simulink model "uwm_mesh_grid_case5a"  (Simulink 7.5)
settings: Solver=ode45  StartTime=0.0  StopTime=3.0  RelTol=1e-4
undefined symbols (not defined in the file or in its folder): D1, Delta, dfilt, DiscIntNeverNeededParam, Discrete, no, powergui, steady, ZData
libraries: powerlib x259, powerlib_extras x68, dsparch4 x11
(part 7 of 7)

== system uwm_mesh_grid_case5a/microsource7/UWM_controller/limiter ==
  In1 : Inport
  Integrator1 : Integrator  LimitOutput=on  UpperSaturationLimit=0  LowerSaturationLimit=-pi  ZeroCross=off
  Integrator2 : Integrator  LimitOutput=on  UpperSaturationLimit=pi  LowerSaturationLimit=0  ZeroCross=off
  Kilim : Gain  Gain=30  ParameterDataType=sfix(16)  ParameterScaling=2^0  OutDataType=sfix(16)  OutScaling=2^0
  Kilim1 : Gain  Gain=30  ParameterDataType=sfix(16)  ParameterScaling=2^0  OutDataType=sfix(16)  OutScaling=2^0
  Kplim : Gain  Gain=3  ParameterDataType=sfix(16)  ParameterScaling=2^0  OutDataType=sfix(16)  OutScaling=2^0
  Kplim1 : Gain  Gain=3  ParameterDataType=sfix(16)  ParameterScaling=2^0  OutDataType=sfix(16)  OutScaling=2^0
  Plimit : Constant  Value=1.0  OutDataType=sfix(16)  OutScaling=2^0
  Plimit1 : Constant  Value=0.0  OutDataType=sfix(16)  OutScaling=2^0
  Saturation1 : Saturate  UpperLimit=pi  LowerLimit=0  OutDataType=fixdt(1, 16)  OutScaling=2^0
  Saturation2 : Saturate  UpperLimit=0  LowerLimit=-pi  OutDataType=fixdt(1, 16)  OutScaling=2^0
  Sum1 : Sum  Inputs=-+|  OutDataType=sfix(16)  OutScaling=2^0
  Sum2 : Sum  Inputs=|++  OutDataType=sfix(16)  OutScaling=2^0
  Sum3 : Sum  OutDataType=sfix(16)  OutScaling=2^0
  Sum4 : Sum  Inputs=|+-  OutDataType=sfix(16)  OutScaling=2^0
  Sum9 : Sum  Inputs=|++  OutDataType=sfix(16)  OutScaling=2^0
  Out1 : Outport
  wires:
  Sum3/1 -> Out1/1
  Plimit1/1 -> Sum1/2
  Integrator2/1 -> Sum2/2
  Kilim1/1 -> Integrator2/1
  Sum1/1 -> Kilim1/1, Kplim1/1
  In1/1 -> Sum1/1, Sum4/2
  Integrator1/1 -> Sum9/2
  Kilim/1 -> Integrator1/1
  Sum4/1 -> Kilim/1, Kplim/1
  Plimit/1 -> Sum4/1
  Kplim1/1 -> Saturation1/1
  Saturation1/1 -> Sum2/1
  Kplim/1 -> Saturation2/1
  Saturation2/1 -> Sum9/1
  Sum9/1 -> Sum3/1
  Sum2/1 -> Sum3/2

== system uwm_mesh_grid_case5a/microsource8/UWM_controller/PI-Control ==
  In1 : Inport
  Gain : Gain  Gain=.01  ParameterDataType=sfix(16)  ParameterScaling=2^0  OutDataType=sfix(16)  OutScaling=2^0
  Gain1 : Gain  Gain=5  ParameterDataType=sfix(16)  ParameterScaling=2^0  OutDataType=sfix(16)  OutScaling=2^0
  Gain2 : Gain  Gain=750  ParameterDataType=sfix(16)  ParameterScaling=2^0  OutDataType=sfix(16)  OutScaling=2^0
  Integrator1 : Integrator  LimitOutput=on  UpperSaturationLimit=100  LowerSaturationLimit=-100  ZeroCross=off
  Sum4 : Sum  Inputs=|++  OutDataType=sfix(16)  OutScaling=2^0
  Out1 : Outport
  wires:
  Gain/1 -> Sum4/1
  Integrator1/1 -> Sum4/2
  In1/1 -> Gain1/1, Gain/1
  Gain1/1 -> Integrator1/1
  Sum4/1 -> Gain2/1
  Gain2/1 -> Out1/1

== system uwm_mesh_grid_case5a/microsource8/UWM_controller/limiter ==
  In1 : Inport
  Integrator1 : Integrator  LimitOutput=on  UpperSaturationLimit=0  LowerSaturationLimit=-pi  ZeroCross=off
  Integrator2 : Integrator  LimitOutput=on  UpperSaturationLimit=pi  LowerSaturationLimit=0  ZeroCross=off
  Kilim : Gain  Gain=30  ParameterDataType=sfix(16)  ParameterScaling=2^0  OutDataType=sfix(16)  OutScaling=2^0
  Kilim1 : Gain  Gain=30  ParameterDataType=sfix(16)  ParameterScaling=2^0  OutDataType=sfix(16)  OutScaling=2^0
  Kplim : Gain  Gain=3  ParameterDataType=sfix(16)  ParameterScaling=2^0  OutDataType=sfix(16)  OutScaling=2^0
  Kplim1 : Gain  Gain=3  ParameterDataType=sfix(16)  ParameterScaling=2^0  OutDataType=sfix(16)  OutScaling=2^0
  Plimit : Constant  Value=1.0  OutDataType=sfix(16)  OutScaling=2^0
  Plimit1 : Constant  Value=0.0  OutDataType=sfix(16)  OutScaling=2^0
  Saturation1 : Saturate  UpperLimit=pi  LowerLimit=0  OutDataType=fixdt(1, 16)  OutScaling=2^0
  Saturation2 : Saturate  UpperLimit=0  LowerLimit=-pi  OutDataType=fixdt(1, 16)  OutScaling=2^0
  Sum1 : Sum  Inputs=-+|  OutDataType=sfix(16)  OutScaling=2^0
  Sum2 : Sum  Inputs=|++  OutDataType=sfix(16)  OutScaling=2^0
  Sum3 : Sum  OutDataType=sfix(16)  OutScaling=2^0
  Sum4 : Sum  Inputs=|+-  OutDataType=sfix(16)  OutScaling=2^0
  Sum9 : Sum  Inputs=|++  OutDataType=sfix(16)  OutScaling=2^0
  Out1 : Outport
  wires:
  Sum3/1 -> Out1/1
  Plimit1/1 -> Sum1/2
  Integrator2/1 -> Sum2/2
  Kilim1/1 -> Integrator2/1
  Sum1/1 -> Kilim1/1, Kplim1/1
  In1/1 -> Sum1/1, Sum4/2
  Integrator1/1 -> Sum9/2
  Kilim/1 -> Integrator1/1
  Sum4/1 -> Kilim/1, Kplim/1
  Plimit/1 -> Sum4/1
  Kplim1/1 -> Saturation1/1
  Saturation1/1 -> Sum2/1
  Kplim/1 -> Saturation2/1
  Saturation2/1 -> Sum9/1
  Sum9/1 -> Sum3/1
  Sum2/1 -> Sum3/2

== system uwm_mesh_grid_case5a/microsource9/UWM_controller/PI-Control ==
  In1 : Inport
  Gain : Gain  Gain=.01  ParameterDataType=sfix(16)  ParameterScaling=2^0  OutDataType=sfix(16)  OutScaling=2^0
  Gain1 : Gain  Gain=5  ParameterDataType=sfix(16)  ParameterScaling=2^0  OutDataType=sfix(16)  OutScaling=2^0
  Gain2 : Gain  Gain=750  ParameterDataType=sfix(16)  ParameterScaling=2^0  OutDataType=sfix(16)  OutScaling=2^0
  Integrator1 : Integrator  LimitOutput=on  UpperSaturationLimit=100  LowerSaturationLimit=-100  ZeroCross=off
  Sum4 : Sum  Inputs=|++  OutDataType=sfix(16)  OutScaling=2^0
  Out1 : Outport
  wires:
  Gain/1 -> Sum4/1
  Integrator1/1 -> Sum4/2
  In1/1 -> Gain1/1, Gain/1
  Gain1/1 -> Integrator1/1
  Sum4/1 -> Gain2/1
  Gain2/1 -> Out1/1

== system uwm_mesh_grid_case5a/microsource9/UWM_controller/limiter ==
  In1 : Inport
  Integrator1 : Integrator  LimitOutput=on  UpperSaturationLimit=0  LowerSaturationLimit=-pi  ZeroCross=off
  Integrator2 : Integrator  LimitOutput=on  UpperSaturationLimit=pi  LowerSaturationLimit=0  ZeroCross=off
  Kilim : Gain  Gain=30  ParameterDataType=sfix(16)  ParameterScaling=2^0  OutDataType=sfix(16)  OutScaling=2^0
  Kilim1 : Gain  Gain=30  ParameterDataType=sfix(16)  ParameterScaling=2^0  OutDataType=sfix(16)  OutScaling=2^0
  Kplim : Gain  Gain=3  ParameterDataType=sfix(16)  ParameterScaling=2^0  OutDataType=sfix(16)  OutScaling=2^0
  Kplim1 : Gain  Gain=3  ParameterDataType=sfix(16)  ParameterScaling=2^0  OutDataType=sfix(16)  OutScaling=2^0
  Plimit : Constant  Value=1.0  OutDataType=sfix(16)  OutScaling=2^0
  Plimit1 : Constant  Value=0.0  OutDataType=sfix(16)  OutScaling=2^0
  Saturation1 : Saturate  UpperLimit=pi  LowerLimit=0  OutDataType=fixdt(1, 16)  OutScaling=2^0
  Saturation2 : Saturate  UpperLimit=0  LowerLimit=-pi  OutDataType=fixdt(1, 16)  OutScaling=2^0
  Sum1 : Sum  Inputs=-+|  OutDataType=sfix(16)  OutScaling=2^0
  Sum2 : Sum  Inputs=|++  OutDataType=sfix(16)  OutScaling=2^0
  Sum3 : Sum  OutDataType=sfix(16)  OutScaling=2^0
  Sum4 : Sum  Inputs=|+-  OutDataType=sfix(16)  OutScaling=2^0
  Sum9 : Sum  Inputs=|++  OutDataType=sfix(16)  OutScaling=2^0
  Out1 : Outport
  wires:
  Sum3/1 -> Out1/1
  Plimit1/1 -> Sum1/2
  Integrator2/1 -> Sum2/2
  Kilim1/1 -> Integrator2/1
  Sum1/1 -> Kilim1/1, Kplim1/1
  In1/1 -> Sum1/1, Sum4/2
  Integrator1/1 -> Sum9/2
  Kilim/1 -> Integrator1/1
  Sum4/1 -> Kilim/1, Kplim/1
  Plimit/1 -> Sum4/1
  Kplim1/1 -> Saturation1/1
  Saturation1/1 -> Sum2/1
  Kplim/1 -> Saturation2/1
  Saturation2/1 -> Sum9/1
  Sum9/1 -> Sum3/1
  Sum2/1 -> Sum3/2

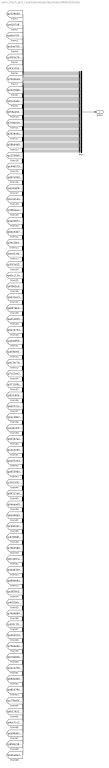
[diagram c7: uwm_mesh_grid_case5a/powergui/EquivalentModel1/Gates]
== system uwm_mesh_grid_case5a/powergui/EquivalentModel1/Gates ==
  Mux : Mux  Inputs=[1 1 1 1 1 1 1 1 1 1 1 1 1 1 1 1 1 1 1 1 1 1 1 1 1 1 1 1 1 1 1 1 1 1 1 1 1 1 1 1 1 1 1 1 1 1 1 1 1 1 1 1 1 1 1 1 1 1 1 1 1 1 1 1 1 1 1 1 1]
  gates : Outport  OutDataType=sfix(16)  OutScaling=2^0
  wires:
  Mux/1 -> gates/1
  [tpe228b584_b106_4beb_8c86_c7c8c8351509] -> Mux/1
  [tpef207a81_30da_459f_9f29_48d5e080c51c] -> Mux/2
  [tpa6e07f33_604f_4639_95d3_65b3053db820] -> Mux/3
  [tpe3ee7652_0b4f_4b52_a6a2_6f5b020b198a] -> Mux/4
  [tp3f93a760_c478_4b19_8b9a_602eaec045ba] -> Mux/5
  [tpfce110a4_06b3_4449_bb13_54bd1c524869] -> Mux/6
  [tp7024ba96_b1e0_402b_98ae_915e2eb8f599] -> Mux/7
  [tp20376989_e36f_4dba_9928_f99e877ec3f8] -> Mux/8
  [tp0ce2ade4_fe95_468c_8653_25d67a2f6720] -> Mux/9
  [tpf56e2625_fa7f_43eb_b96b_8aa41f0e0eb0] -> Mux/10
  [tp7c8d1b9a_a0ac_4205_9121_39a3ef8997d4] -> Mux/11
  [tp2628d4ad_802e_4e1e_86c6_7d3f78e79741] -> Mux/12
  [tp58b64b92_acf2_4221_8757_7d28af085dd6] -> Mux/13
  [tpc5536b6e_0140_4226_96f4_1f886dbf2188] -> Mux/14
  [tpc446579b_ad45_4666_855e_414268daf5d6] -> Mux/15
  [tpd07e0087_c4a6_4b78_9156_ac2b3f1b5b6f] -> Mux/16
  [tpda5a6f64_d918_47c0_b755_b8f491cd819e] -> Mux/17
  [tp5c2e14aa_08b7_47f7_8143_25f87816b941] -> Mux/18
  [tp79bdace3_b7b0_4249_b087_69f27f13bbc9] -> Mux/19
  [tp4a02671c_43fe_4e01_980c_0eab1f5b6319] -> Mux/20
  [tp0deddd7d_a945_4a8b_8921_7258e67777da] -> Mux/21
  [tp3ec2bb15_666f_445f_a31f_f1abb802b23d] -> Mux/22
  [tpaee1afd5_2a3a_4c4e_81d1_932180aaf4cd] -> Mux/23
  [tp35f3d32d_77d0_4ec4_8380_fc1713e814fd] -> Mux/24
  [tpd5cc13b4_db93_4301_a375_bb18755ebe77] -> Mux/25
  [tpf4062e95_3443_47db_82c0_350cf0c25750] -> Mux/26
  [tp9531e23f_24be_4071_8584_f51bbd60ef4e] -> Mux/27
  [tp69f76bb8_fdbd_4204_8031_d9110d10a512] -> Mux/28
  [tpad1e850b_84d7_4b4f_84eb_080e44351dad] -> Mux/29
  [tpbb747444_63b8_44b4_b818_e0e58927764a] -> Mux/30
  [tp1b44f6bb_f2da_48c5_bb83_4960df7e179a] -> Mux/31
  [tpb5fb0f4c_cf62_4fd9_80a4_68c4b2356418] -> Mux/32
  [tpdc3ec7bb_0663_4ba0_89e4_c1c6bfdf648e] -> Mux/33
  [tp7c52ee29_3c12_4bfa_b7a2_65a1122460f4] -> Mux/34
  [tp371168cb_fc82_4ba0_b16c_c880a08d5024] -> Mux/35
  [tp62fc80bf_2011_4d5e_9be1_b2d6273b3ea2] -> Mux/36
  [tpbd0721ef_db8d_47f7_9890_7defe1fe666e] -> Mux/37
  [tp53c38974_2706_42db_94c7_ddd4e4d3b246] -> Mux/38
  [tp1a6c43fb_a676_4586_a0d1_c5ff8f0d4ae2] -> Mux/39
  [tp933b7aeb_9fdc_4218_80c6_68c9129134d2] -> Mux/40
  [tp13e31956_19c2_465e_9930_ef33d808f5d3] -> Mux/41
  [tpaa07ae4e_8a98_4286_a633_7e0dd46b920b] -> Mux/42
  [tpa65396d1_e5c2_4e4a_8dcb_8dd232d9dcff] -> Mux/43
  [tp7817f936_9030_445a_b91d_d11df62fcea4] -> Mux/44
  [tp84221b66_9ec3_426a_9c58_687200c2f280] -> Mux/45
  [tp5deead94_68b6_4323_ad82_4c4e3d7e236e] -> Mux/46
  [tp8aa98edc_83de_43f3_b92f_8a5361184f9a] -> Mux/47
  [tpc9002618_045e_4d6a_ac72_a68281a96bd7] -> Mux/48
  [tp673f69f6_82ca_4338_aa87_d59190bf68bf] -> Mux/49
  [tp7bb55887_ef87_424a_af1b_5f1901cf865a] -> Mux/50
  [tp6c446ce2_6cd8_46c3_9120_bda7217b6b5f] -> Mux/51
  [tpd4dd329b_3e2b_4ba8_9125_5a1fe0d0b51a] -> Mux/52
  [tpd69eb8ae_aeda_4526_9dd4_f402d4137f04] -> Mux/53
  [tpc605fb3f_fb8c_4d73_b613_a089dad69b67] -> Mux/54
  [tp4f07b6c9_f4fc_449c_8932_a78d658e8135] -> Mux/55
  [tp74d68840_4b65_4268_ba1a_ab971938b5e8] -> Mux/56
  [tp592c1fc9_f3c2_44fd_b305_e35d9eb2ac04] -> Mux/57
  [tpa5b5019c_88d7_4d6f_9ab7_8e2d3a81cd78] -> Mux/58
  [tp75bde6a7_ec4d_4fc1_be1b_a4b562858042] -> Mux/59
  [tp0c5bb0bd_c4ad_4771_9dea_76c1bb1f8057] -> Mux/60
  [tp2ec27d90_4684_4437_8959_f6e479ef260b] -> Mux/61
  [tpb8dbdd89_c217_41ad_bcb2_15a8ca9ae5c1] -> Mux/62
  [tpe81079eb_0f20_43dd_885d_1225b6d7928e] -> Mux/63
  [tpc79ed3fe_559f_4f8f_be41_c95cc4f1d8e1] -> Mux/64
  [tpfb178219_10dc_471f_9f4e_2f5eeda652e1] -> Mux/65
  [tp4ac7cc24_7bdd_464e_9199_ae2da14c3347] -> Mux/66
  [tpee96da57_8a75_4e0e_8896_4195514b6dd0] -> Mux/67
  [tp9f48c58f_8624_4c9f_89d7_eb94e2365c4b] -> Mux/68
  [tp52be8a3f_5ef1_470d_9c61_385db7766b04] -> Mux/69

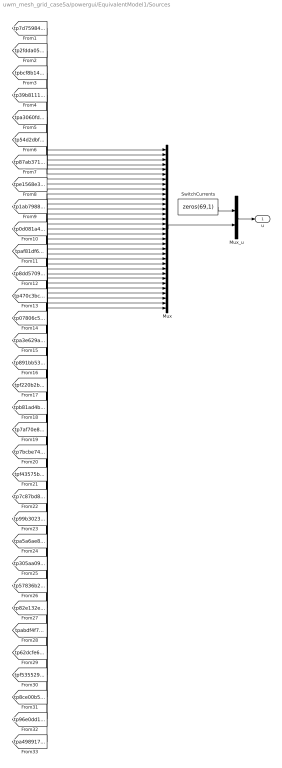
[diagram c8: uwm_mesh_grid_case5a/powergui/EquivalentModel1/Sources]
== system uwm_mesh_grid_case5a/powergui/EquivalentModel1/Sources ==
  Mux : Mux  Inputs=[2 2 1 1 1 1 1 1 1 1 1 1 1 1 1 1 1 1 1 1 1 1 1 1 1 1 1 1 1 1 1 1 3]
  Mux_u : Mux  Inputs=[69 37]
  SwitchCurrents : Constant  Value=zeros(69,1)  OutDataType=sfix(16)  OutScaling=2^0
  u : Outport  OutDataType=sfix(16)  OutScaling=2^0
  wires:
  Mux/1 -> Mux_u/2
  SwitchCurrents/1 -> Mux_u/1
  Mux_u/1 -> u/1
  [tp7d759843_31d9_4042_9dd1_9d642f5f0ff6] -> Mux/1
  [tp2fdda057_d641_4494_87e2_4c9b57d21964] -> Mux/2
  [tpbcf8b145_bdbd_45a5_8180_c3b948527696] -> Mux/3
  [tp39b81111_6fe0_4f05_ad16_780e8486a916] -> Mux/4
  [tpa3060fd9_7bb9_417d_8175_8f81b43b5773] -> Mux/5
  [tp54d2dbf4_60ce_493f_bb15_bc46fa13cfce] -> Mux/6
  [tp87ab3716_8e1d_4485_9e1a_7dc248724a34] -> Mux/7
  [tpe1568e33_bb97_4973_8708_9b1bfa17e7b5] -> Mux/8
  [tp1ab79880_228a_47d9_b201_2eba8816ee37] -> Mux/9
  [tp0d081a4d_5e9f_4b80_b4bf_20152486f853] -> Mux/10
  [tpaf81df68_c781_4da9_928a_44e197fbd618] -> Mux/11
  [tp8dd5709b_0ddf_41b6_8112_b238b0604763] -> Mux/12
  [tp470c3bc4_f7fa_46bc_9d1d_7daedd95ab4d] -> Mux/13
  [tp07806c5c_c32f_4993_b5c9_0567717f058b] -> Mux/14
  [tpa3e629a0_aa84_4358_8c69_1a4ec5cc445c] -> Mux/15
  [tp891bb538_b5bf_4ed0_b431_af5b4feecf62] -> Mux/16
  [tpf220b2bc_30ec_49dc_84aa_16925a585808] -> Mux/17
  [tpb81ad4b4_5942_43b4_8611_4a5e3db6afea] -> Mux/18
  [tp7af70e86_5434_4a0b_a65f_cb50f4951e25] -> Mux/19
  [tp7bcbe742_1608_4799_b18e_3f319801db3a] -> Mux/20
  [tpf43575be_15e6_453b_8afc_ade3ef51566d] -> Mux/21
  [tp7c87bd8b_32e3_4f6e_b2e4_4d41421fbded] -> Mux/22
  [tp99b3023c_53a1_4cb1_8eb9_8a0dd0b275b4] -> Mux/23
  [tpa5a6ae8e_c854_40e8_9ddc_396f1146314e] -> Mux/24
  [tp305aa09b_c490_428b_885a_4fbc8d6842c6] -> Mux/25
  [tp57836b25_c200_437c_8731_9b11c5d96589] -> Mux/26
  [tp82e132eb_2e2c_4493_9e5a_5b60972280db] -> Mux/27
  [tpabdf4f74_f4c9_43eb_b6bb_d288b3c0828e] -> Mux/28
  [tp62dcfe63_a088_4110_93e8_40b42f148094] -> Mux/29
  [tpf535529d_f631_44eb_ab48_591eb2ee78c0] -> Mux/30
  [tp8ce00b5d_5cb0_4337_89a4_c9ddeba94b1d] -> Mux/31
  [tp96e0dd11_cb3a_442d_8983_7206ff209956] -> Mux/32
  [tpa4989172_9284_44b3_847a_72b6f9fc12e1] -> Mux/33

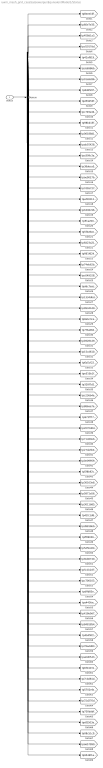
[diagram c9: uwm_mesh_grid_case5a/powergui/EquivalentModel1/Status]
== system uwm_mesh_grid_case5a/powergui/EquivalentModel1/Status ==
  status : Inport  OutDataType=sfix(16)  OutScaling=2^0
  Demux : Demux  Outputs=[1 1 1 1 1 1 1 1 1 1 1 1 1 1 1 1 1 1 1 1 1 1 1 1 1 1 1 1 1 1 1 1 1 1 1 1 1 1 1 1 1 1 1 1 1 1 1 1 1 1 1 1 1 1 1 1 1 1 1 1 1 1 1 1 1 1 1 1 1]
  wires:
  status/1 -> Demux/1
  Demux/1 -> [tp8eee16f0_73bc_426a_923f_d0f8c13bafd5]
  Demux/2 -> [tp60e7e35c_5f12_4a0e_9718_b32ce2ba50d0]
  Demux/3 -> [tp458d1a33_cda1_4594_b291_3037858a6a3d]
  Demux/4 -> [tpd1017dd6_fe52_43e1_9e32_9a82b07cf3e7]
  Demux/5 -> [tp42af919c_2b93_4996_b563_63afbb6576d1]
  Demux/6 -> [tpc66986b1_bd46_431e_955a_89d3e209ef11]
  Demux/7 -> [tp01a9d368_bc66_4568_b999_b99960807b75]
  Demux/8 -> [tp8d6f20f4_9270_4a74_9e34_5e801ba0a5c9]
  Demux/9 -> [tpd59d50fe_f10d_45b9_a176_da10036f4416]
  Demux/10 -> [tpc749e44d_193e_4184_abf1_a8a792175895]
  Demux/11 -> [tp98bb15f7_383f_4745_afda_771091a7a65a]
  Demux/12 -> [tp00188d10_d74e_488c_9cfc_e0d01f9d8f24]
  Demux/13 -> [tpab55428f_5349_40a0_9716_b4957136b2bc]
  Demux/14 -> [tpa309c3a8_bbb7_406b_9ab7_3101dc644993]
  Demux/15 -> [tp38abca51_76f8_4f01_9ce1_f260d733e2bb]
  Demux/16 -> [tpae0027b8_727e_4109_ad78_625216868f53]
  Demux/17 -> [tp7db5727d_1a32_4102_a8a0_12c3d22a2e02]
  Demux/18 -> [tpaf202125_9f29_4d88_b2d2_8ef4cef4b279]
  Demux/19 -> [tp6306c964_1d11_410b_86c0_fef2c1c4967c]
  Demux/20 -> [tpffca200e_48e5_4844_9425_4274ee627a54]
  Demux/21 -> [tp5f4a9ee5_318c_496c_8536_e76be5b8a50d]
  Demux/22 -> [tp6d23a21c_2996_43b3_b136_db87cecd02fb]
  Demux/23 -> [tp961f6248_70f3_4c5e_aaee_3103c04ab32e]
  Demux/24 -> [tp74eb62b7_47ae_4708_ab69_5a92f2a1414a]
  Demux/25 -> [tpc0493283_7478_4a22_85a7_451f8bed842a]
  Demux/26 -> [tpddc7eac8_8c8c_4e8a_8602_688544ef6d33]
  Demux/27 -> [tp1334dbd4_7809_4f73_9c14_f9d87e14eae4]
  Demux/28 -> [tp99341d9c_9317_4298_b5f6_bf74b15c98eb]
  Demux/29 -> [tp8ebc3cea_b386_4b0e_880e_2e608cb19e20]
  Demux/30 -> [tp7f3a6840_09e1_41bf_be4e_6c6f6a1ae37a]
  Demux/31 -> [tpb9281d9c_0afb_4ca2_87e9_9bcc785ce5b5]
  Demux/32 -> [tp15cd6109_61ac_45ed_bd45_891a2b62bd3c]
  Demux/33 -> [tp6a5cf22c_b669_4f6e_8633_cc44e782f77f]
  Demux/34 -> [tpe510b1f0_593f_480f_89d5_de2155ea611a]
  Demux/35 -> [tp328f7d2e_9f35_43ce_803f_8ac94d8a7cd6]
  Demux/36 -> [tpc236b4a1_a8e8_46ce_b518_21694a0dc189]
  Demux/37 -> [tp886ae7a3_4fe7_4310_96e6_b93d749dbaff]
  Demux/38 -> [tp972ff777_56b8_46b3_ba85_e8929cc69bdd]
  Demux/39 -> [tp2070d6d7_60f3_4435_9da0_5593a767a846]
  Demux/40 -> [tp71d40eb9_664b_4b11_ad0f_fbc7c4113756]
  Demux/41 -> [tp27da3b4f_eef3_4dc2_a2cf_cf4a6727acbf]
  Demux/42 -> [tp0e099590_86aa_4462_816f_0eff386a13bf]
  Demux/43 -> [tp5f8b92cd_5788_4f99_954a_5e37a7a36027]
  Demux/44 -> [tp30163e8d_1663_4dfc_b77f_820804da0d80]
  Demux/45 -> [tp5871a565_e56f_42c6_a674_003f612766d6]
  Demux/46 -> [tp3011b85c_3f40_40c6_a00c_5fcb9e864164]
  Demux/47 -> [tp41fc1d8e_28c5_4f8c_b557_161b91bb1cf2]
  Demux/48 -> [tpd9816bb9_0a79_4196_8804_998df722d2ba]
  Demux/49 -> [tpff890369_a8a2_4d9f_a089_7f10d53e1578]
  Demux/50 -> [tp5d5bd247_6b92_46da_97fc_cd62913ed9c8]
  Demux/51 -> [tp9eb67400_5185_47c4_b94f_301d2b76785b]
  Demux/52 -> [tp5c1b2d7f_46dd_49bf_ac53_56b184fb2616]
  Demux/53 -> [tpc7001033_01c3_40f1_bbff_62eed500eaf9]
  Demux/54 -> [tpdffb83e0_a436_4b15_bd15_19f107b484b9]
  Demux/55 -> [tpa443fac7_c9b5_4684_b9c0_75e06020489c]
  Demux/56 -> [tp418e9d76_d26f_4f97_b6e4_dba7cf226ef7]
  Demux/57 -> [tp84818548_693f_4034_8abd_404ceec9c271]
  Demux/58 -> [tp4b4f4f2c_262d_4226_8d2c_f54a81e0f973]
  Demux/59 -> [tp78add83b_5514_4b69_b9e3_5c5b550847b4]
  Demux/60 -> [tpa6d0543d_ca1e_4bf3_bdf1_667ac18f1547]
  Demux/61 -> [tp6f242312_db03_47aa_8437_0a78a23077f8]
  Demux/62 -> [tp7cbd81d6_b469_4dba_a454_39d50f6b7e04]
  Demux/63 -> [tp5702efad_dab6_4069_bd4b_bd74550e3e40]
  Demux/64 -> [tp31d270da_e899_4935_9399_84cbfd39a9ef]
  Demux/65 -> [tp730dddf7_4db6_4a1e_94b5_093b926c693e]
  Demux/66 -> [tpdf2503ab_0cb6_4d0c_a681_b772a7c3afc4]
  Demux/67 -> [tp08c51c09_df2f_4d94_8299_f53cae399876]
  Demux/68 -> [tpa6579907_d096_4778_a593_7ecda243f049]
  Demux/69 -> [tp9546f1a8_826f_4cf4_8ef3_e912cb27772c]

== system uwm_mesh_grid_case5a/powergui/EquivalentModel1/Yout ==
  v,i : Inport  OutDataType=sfix(16)  OutScaling=2^0
  Demux : Demux  Outputs=[202 120]
  sub1 : Subsystem
  sub2 : Subsystem
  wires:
  v,i/1 -> Demux/1
  Demux/1 -> sub1/1(input)
  Demux/2 -> sub2/1(input)

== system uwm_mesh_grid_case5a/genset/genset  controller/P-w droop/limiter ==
  In1 : Inport
  Integrator1 : Integrator  UpperSaturationLimit=0  LowerSaturationLimit=-2*pi
  Integrator2 : Integrator  UpperSaturationLimit=2*pi  LowerSaturationLimit=0
  Kilim : Gain  Gain=30  ParameterDataType=sfix(16)  ParameterScaling=2^0  OutDataType=sfix(16)  OutScaling=2^0
  Kilim1 : Gain  Gain=30  ParameterDataType=sfix(16)  ParameterScaling=2^0  OutDataType=sfix(16)  OutScaling=2^0
  Kilim2 : Gain  ParameterDataType=sfix(16)  ParameterScaling=2^0  OutDataType=sfix(16)  OutScaling=2^0
  Kilim3 : Gain  ParameterDataType=sfix(16)  ParameterScaling=2^0  OutDataType=sfix(16)  OutScaling=2^0
  Kilim4 : Gain  ParameterDataType=sfix(16)  ParameterScaling=2^0  OutDataType=sfix(16)  OutScaling=2^0
  Kplim : Gain  Gain=3  ParameterDataType=sfix(16)  ParameterScaling=2^0  OutDataType=sfix(16)  OutScaling=2^0
  Kplim1 : Gain  Gain=3  ParameterDataType=sfix(16)  ParameterScaling=2^0  OutDataType=sfix(16)  OutScaling=2^0
  Plimit : Constant  Value=1.0  OutDataType=sfix(16)  OutScaling=2^0
  Plimit1 : Constant  Value=0.0  OutDataType=sfix(16)  OutScaling=2^0
  Saturation1 : Saturate  UpperLimit=pi  LowerLimit=0  OutDataType=fixdt(1, 16)  OutScaling=2^0
  Saturation2 : Saturate  UpperLimit=0  LowerLimit=-pi  OutDataType=fixdt(1, 16)  OutScaling=2^0
  Sum1 : Sum  Inputs=-+|  OutDataType=sfix(16)  OutScaling=2^0
  Sum2 : Sum  Inputs=|++  OutDataType=sfix(16)  OutScaling=2^0
  Sum3 : Sum  OutDataType=sfix(16)  OutScaling=2^0
  Sum4 : Sum  Inputs=|+-  OutDataType=sfix(16)  OutScaling=2^0
  Sum9 : Sum  Inputs=|++  OutDataType=sfix(16)  OutScaling=2^0
  Out1 : Outport
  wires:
  Sum3/1 -> Out1/1
  Saturation2/1 -> Sum3/1
  Saturation1/1 -> Sum3/2
  Sum2/1 -> Saturation1/1
  Integrator2/1 -> Sum2/2
  Kplim1/1 -> Sum2/1
  Kilim1/1 -> Integrator2/1
  Sum1/1 -> Kilim1/1, Kplim1/1
  Sum9/1 -> Saturation2/1
  Integrator1/1 -> Sum9/2
  Kplim/1 -> Sum9/1
  Kilim/1 -> Integrator1/1
  Sum4/1 -> Kilim/1, Kplim/1
  Kilim2/1 -> Sum4/1
  Plimit/1 -> Kilim2/1
  In1/1 -> Kilim3/1
  Kilim3/1 -> Sum4/2, Sum1/1
  Plimit1/1 -> Kilim4/1
  Kilim4/1 -> Sum1/2

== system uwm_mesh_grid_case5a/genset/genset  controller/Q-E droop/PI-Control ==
  In1 : Inport
  Constant1 : Constant  OutDataType=fixdt(1, 16)  OutScaling=2^0
  Gain : Gain  Gain=1000  ParameterDataType=sfix(16)  ParameterScaling=2^0  OutDataType=sfix(16)  OutScaling=2^0
  Gain1 : Gain  Gain=10  ParameterDataType=sfix(16)  ParameterScaling=2^0  OutDataType=sfix(16)  OutScaling=2^0
  Integrator1 : Integrator  InitialCondition=.88  UpperSaturationLimit=1  LowerSaturationLimit=-1
  Sum1 : Sum  Inputs=|++  OutDataType=sfix(16)  OutScaling=2^0
  Sum4 : Sum  Inputs=|++  OutDataType=sfix(16)  OutScaling=2^0
  Out1 : Outport
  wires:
  Gain/1 -> Sum4/1
  Integrator1/1 -> Sum4/2
  In1/1 -> Gain1/1, Gain/1
  Gain1/1 -> Integrator1/1
  Sum1/1 -> Out1/1
  Sum4/1 -> Sum1/1
  Constant1/1 -> Sum1/2

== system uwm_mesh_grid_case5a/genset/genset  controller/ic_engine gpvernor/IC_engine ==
  fuel_cmd : Inport  OutDataType=fixdt(1, 16)  OutScaling=2^0
  wr : Inport  Port=2  OutDataType=fixdt(1, 16)  OutScaling=2^0
  Delay : TransportDelay  DelayTime=.022
  Friction_losses : Fcn  Expr=u(1)*u(1)*u(2)
  Fuel_torque : Fcn  Expr=u(1)*3.6*11.8238*0.47*1000
  Mux : Mux  Inputs=2
  Mux1 : Mux  Inputs=2
  Power Limit : Saturate  UpperLimit=1  LowerLimit=0  OutDataType=fixdt(1, 16)  OutScaling=2^0
  Sum : Sum  Inputs=|+-  OutDataType=fixdt(1, 16)  OutScaling=2^0
  Torque_to_power_pu : Fcn  Expr=u(1)*u(2)/12500
  mech_losses : Constant  Value=0.36  OutDataType=fixdt(1, 16)  OutScaling=2^0
  Pmech : Outport  OutDataType=fixdt(1, 16)  OutScaling=2^0
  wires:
  Fuel_torque/1 -> Delay/1
  fuel_cmd/1 -> Fuel_torque/1
  Delay/1 -> Mux/1
  wr/1 -> Mux/2, Mux1/1
  mech_losses/1 -> Mux1/2
  Mux1/1 -> Friction_losses/1
  Mux/1 -> Torque_to_power_pu/1
  Torque_to_power_pu/1 -> Sum/1
  Friction_losses/1 -> Sum/2
  Sum/1 -> Power Limit/1
  Power Limit/1 -> Pmech/1

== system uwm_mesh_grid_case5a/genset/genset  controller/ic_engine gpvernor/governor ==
  Pmeas : Inport  OutDataType=fixdt(1, 16)  OutScaling=2^0
  w : Inport  Port=2  OutDataType=fixdt(1, 16)  OutScaling=2^0
  wr : Inport  Port=3  OutDataType=fixdt(1, 16)  OutScaling=2^0
  Gain : Gain  Gain=20  ParameterDataType=fixdt(1, 16)  ParameterScaling=2^0  OutDataType=fixdt(1, 16)  OutScaling=2^0
  Gain1 : Gain  Gain=10  ParameterDataType=fixdt(1, 16)  ParameterScaling=2^0  OutDataType=fixdt(1, 16)  OutScaling=2^0
  Integrator : Integrator  LimitOutput=on  UpperSaturationLimit=10  LowerSaturationLimit=-10
  Sum : Sum  Inputs=-+|  OutDataType=fixdt(1, 16)  OutScaling=2^0
  Sum1 : Sum  Inputs=++|  OutDataType=fixdt(1, 16)  OutScaling=2^0
  Sum2 : Sum  Inputs=++|  OutDataType=fixdt(1, 16)  OutScaling=2^0
  Te_cmd_t0_fuel : Fcn  Expr=u(1)/1.6
  Torque_limit : Saturate  UpperLimit=1000  LowerLimit=-1000  OutDataType=fixdt(1, 16)  OutScaling=2^0
  fuel_cmd : Outport  OutDataType=fixdt(1, 16)  OutScaling=2^0
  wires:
  w/1 -> Sum/2
  wr/1 -> Sum/1
  Sum/1 -> Integrator/1, Gain1/1
  Integrator/1 -> Gain/1
  Gain/1 -> Sum1/1
  Gain1/1 -> Sum1/2
  Pmeas/1 -> Sum2/1
  Sum1/1 -> Sum2/2
  Sum2/1 -> Torque_limit/1
  Torque_limit/1 -> Te_cmd_t0_fuel/1
  Te_cmd_t0_fuel/1 -> fuel_cmd/1

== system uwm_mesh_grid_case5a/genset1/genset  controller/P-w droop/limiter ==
  In1 : Inport
  Integrator1 : Integrator  UpperSaturationLimit=0  LowerSaturationLimit=-2*pi
  Integrator2 : Integrator  UpperSaturationLimit=2*pi  LowerSaturationLimit=0
  Kilim : Gain  Gain=30  ParameterDataType=sfix(16)  ParameterScaling=2^0  OutDataType=sfix(16)  OutScaling=2^0
  Kilim1 : Gain  Gain=30  ParameterDataType=sfix(16)  ParameterScaling=2^0  OutDataType=sfix(16)  OutScaling=2^0
  Kilim2 : Gain  ParameterDataType=sfix(16)  ParameterScaling=2^0  OutDataType=sfix(16)  OutScaling=2^0
  Kilim3 : Gain  ParameterDataType=sfix(16)  ParameterScaling=2^0  OutDataType=sfix(16)  OutScaling=2^0
  Kilim4 : Gain  ParameterDataType=sfix(16)  ParameterScaling=2^0  OutDataType=sfix(16)  OutScaling=2^0
  Kplim : Gain  Gain=3  ParameterDataType=sfix(16)  ParameterScaling=2^0  OutDataType=sfix(16)  OutScaling=2^0
  Kplim1 : Gain  Gain=3  ParameterDataType=sfix(16)  ParameterScaling=2^0  OutDataType=sfix(16)  OutScaling=2^0
  Plimit : Constant  Value=1.0  OutDataType=sfix(16)  OutScaling=2^0
  Plimit1 : Constant  Value=0.0  OutDataType=sfix(16)  OutScaling=2^0
  Saturation1 : Saturate  UpperLimit=pi  LowerLimit=0  OutDataType=fixdt(1, 16)  OutScaling=2^0
  Saturation2 : Saturate  UpperLimit=0  LowerLimit=-pi  OutDataType=fixdt(1, 16)  OutScaling=2^0
  Sum1 : Sum  Inputs=-+|  OutDataType=sfix(16)  OutScaling=2^0
  Sum2 : Sum  Inputs=|++  OutDataType=sfix(16)  OutScaling=2^0
  Sum3 : Sum  OutDataType=sfix(16)  OutScaling=2^0
  Sum4 : Sum  Inputs=|+-  OutDataType=sfix(16)  OutScaling=2^0
  Sum9 : Sum  Inputs=|++  OutDataType=sfix(16)  OutScaling=2^0
  Out1 : Outport
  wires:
  Sum3/1 -> Out1/1
  Saturation2/1 -> Sum3/1
  Saturation1/1 -> Sum3/2
  Sum2/1 -> Saturation1/1
  Integrator2/1 -> Sum2/2
  Kplim1/1 -> Sum2/1
  Kilim1/1 -> Integrator2/1
  Sum1/1 -> Kilim1/1, Kplim1/1
  Sum9/1 -> Saturation2/1
  Integrator1/1 -> Sum9/2
  Kplim/1 -> Sum9/1
  Kilim/1 -> Integrator1/1
  Sum4/1 -> Kilim/1, Kplim/1
  Kilim2/1 -> Sum4/1
  Plimit/1 -> Kilim2/1
  In1/1 -> Kilim3/1
  Kilim3/1 -> Sum4/2, Sum1/1
  Plimit1/1 -> Kilim4/1
  Kilim4/1 -> Sum1/2

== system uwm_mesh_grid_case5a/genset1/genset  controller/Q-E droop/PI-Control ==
  In1 : Inport
  Constant1 : Constant  OutDataType=fixdt(1, 16)  OutScaling=2^0
  Gain : Gain  Gain=1000  ParameterDataType=sfix(16)  ParameterScaling=2^0  OutDataType=sfix(16)  OutScaling=2^0
  Gain1 : Gain  Gain=10  ParameterDataType=sfix(16)  ParameterScaling=2^0  OutDataType=sfix(16)  OutScaling=2^0
  Integrator1 : Integrator  InitialCondition=.88  UpperSaturationLimit=1  LowerSaturationLimit=-1
  Sum1 : Sum  Inputs=|++  OutDataType=sfix(16)  OutScaling=2^0
  Sum4 : Sum  Inputs=|++  OutDataType=sfix(16)  OutScaling=2^0
  Out1 : Outport
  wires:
  Gain/1 -> Sum4/1
  Integrator1/1 -> Sum4/2
  In1/1 -> Gain1/1, Gain/1
  Gain1/1 -> Integrator1/1
  Sum1/1 -> Out1/1
  Sum4/1 -> Sum1/1
  Constant1/1 -> Sum1/2

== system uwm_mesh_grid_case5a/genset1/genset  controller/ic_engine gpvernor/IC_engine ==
  fuel_cmd : Inport  OutDataType=fixdt(1, 16)  OutScaling=2^0
  wr : Inport  Port=2  OutDataType=fixdt(1, 16)  OutScaling=2^0
  Delay : TransportDelay  DelayTime=.022
  Friction_losses : Fcn  Expr=u(1)*u(1)*u(2)
  Fuel_torque : Fcn  Expr=u(1)*3.6*11.8238*0.47*1000
  Mux : Mux  Inputs=2
  Mux1 : Mux  Inputs=2
  Power Limit : Saturate  UpperLimit=1  LowerLimit=0  OutDataType=fixdt(1, 16)  OutScaling=2^0
  Sum : Sum  Inputs=|+-  OutDataType=fixdt(1, 16)  OutScaling=2^0
  Torque_to_power_pu : Fcn  Expr=u(1)*u(2)/12500
  mech_losses : Constant  Value=0.36  OutDataType=fixdt(1, 16)  OutScaling=2^0
  Pmech : Outport  OutDataType=fixdt(1, 16)  OutScaling=2^0
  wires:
  Fuel_torque/1 -> Delay/1
  fuel_cmd/1 -> Fuel_torque/1
  Delay/1 -> Mux/1
  wr/1 -> Mux/2, Mux1/1
  mech_losses/1 -> Mux1/2
  Mux1/1 -> Friction_losses/1
  Mux/1 -> Torque_to_power_pu/1
  Torque_to_power_pu/1 -> Sum/1
  Friction_losses/1 -> Sum/2
  Sum/1 -> Power Limit/1
  Power Limit/1 -> Pmech/1

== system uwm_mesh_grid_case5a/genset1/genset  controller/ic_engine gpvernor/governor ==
  Pmeas : Inport  OutDataType=fixdt(1, 16)  OutScaling=2^0
  w : Inport  Port=2  OutDataType=fixdt(1, 16)  OutScaling=2^0
  wr : Inport  Port=3  OutDataType=fixdt(1, 16)  OutScaling=2^0
  Gain : Gain  Gain=20  ParameterDataType=fixdt(1, 16)  ParameterScaling=2^0  OutDataType=fixdt(1, 16)  OutScaling=2^0
  Gain1 : Gain  Gain=10  ParameterDataType=fixdt(1, 16)  ParameterScaling=2^0  OutDataType=fixdt(1, 16)  OutScaling=2^0
  Integrator : Integrator  LimitOutput=on  UpperSaturationLimit=10  LowerSaturationLimit=-10
  Sum : Sum  Inputs=-+|  OutDataType=fixdt(1, 16)  OutScaling=2^0
  Sum1 : Sum  Inputs=++|  OutDataType=fixdt(1, 16)  OutScaling=2^0
  Sum2 : Sum  Inputs=++|  OutDataType=fixdt(1, 16)  OutScaling=2^0
  Te_cmd_t0_fuel : Fcn  Expr=u(1)/1.6
  Torque_limit : Saturate  UpperLimit=1000  LowerLimit=-1000  OutDataType=fixdt(1, 16)  OutScaling=2^0
  fuel_cmd : Outport  OutDataType=fixdt(1, 16)  OutScaling=2^0
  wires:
  w/1 -> Sum/2
  wr/1 -> Sum/1
  Sum/1 -> Integrator/1, Gain1/1
  Integrator/1 -> Gain/1
  Gain/1 -> Sum1/1
  Gain1/1 -> Sum1/2
  Pmeas/1 -> Sum2/1
  Sum1/1 -> Sum2/2
  Sum2/1 -> Torque_limit/1
  Torque_limit/1 -> Te_cmd_t0_fuel/1
  Te_cmd_t0_fuel/1 -> fuel_cmd/1

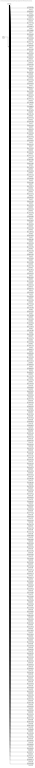
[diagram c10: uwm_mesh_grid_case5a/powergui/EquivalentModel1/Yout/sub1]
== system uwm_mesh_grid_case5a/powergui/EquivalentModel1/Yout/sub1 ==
  input : Inport  OutDataType=sfix(16)  OutScaling=2^0
  Demux : Demux  Outputs=[1 1 1 1 1 1 1 1 1 1 1 1 1 1 1 1 1 1 1 1 1 1 1 1 1 1 1 1 1 1 1 1 1 1 1 1 1 1 1 1 1 1 1 1 1 1 1 1 1 1 1 1 1 1 1 1 1 1 1 1 1 1 1 1 1 1 1 1 1 2 2 1 1 1 1 1 1 1 1 1 1 1 1 1 1 1 1 1 1 1 1 1 1 1 1 1 1 1 1 1 1 1 1 1 1 1 1 1 1 1 1 1 1 1 1 1 1 1 1 1 1 1 1 1 1 1 1 1 1 1 1 1 1 1 1 1 1 1 1 1 1 1 1 1 1 1 1 1 1 1 1 1 1 1 1 1 1 1 1 1 1 1 1 1 1 1 1 1 1 1 1 1 1 1 1 1 1 1 1 1 1 1 1 1 1 1 1 1 1 1 1 1 1 1 1 1 1 1 1 1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
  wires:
  input/1 -> Demux/1
  Demux/1 -> [tpd5b188db_283e_4cef_9afd_4dd5c94b0fec]
  Demux/2 -> [tp0189eff7_d497_4b95_83d8_43ca3fe7c6ed]
  Demux/3 -> [tp1d4d063b_1eb4_49ac_836a_091045dec02e]
  Demux/4 -> [tp0cf022ce_17b0_48f9_ae13_d33fc3a73abd]
  Demux/5 -> [tp374b775e_03b7_40e5_af86_2658eb8c8798]
  Demux/6 -> [tpf1dfb411_d6b8_48a7_bde0_53f33f32148b]
  Demux/7 -> [tpcb18806c_7b44_4c72_8752_eff13f4131a5]
  Demux/8 -> [tp1d4eeda4_6360_4e01_8826_28fca96372eb]
  Demux/9 -> [tp5bd39a8a_a4fd_43da_ae9f_3c385d0365e6]
  Demux/10 -> [tpd4c2771b_c8bb_45ae_8bdf_1cce51ac689a]
  Demux/11 -> [tpa09fad9a_7875_4b05_a164_018d82629fd1]
  Demux/12 -> [tp4c7c1624_1b4f_4d32_914a_db9a7e8368d1]
  Demux/13 -> [tpb7e78c4d_d9e0_4d70_ae87_69151746d2c8]
  Demux/14 -> [tp6f683f83_0832_4c84_b035_fd827a547197]
  Demux/15 -> [tpfb9aca37_00d1_4425_a403_7465db9239ad]
  Demux/16 -> [tpa0d3a7bd_5845_4ae6_a892_688a497819f4]
  Demux/17 -> [tp72469e22_ec1c_452f_af42_fea3f395c65d]
  Demux/18 -> [tpc9b65cda_f631_445b_bd77_145c0cb57b53]
  Demux/19 -> [tpa58dbed4_d424_438a_88a9_1b0cdd51dd8c]
  Demux/20 -> [tp6a93cd57_9a4e_45f4_98f9_25b091282e28]
  Demux/21 -> [tpeb53911a_00be_440f_93a1_59a8914e49f2]
  Demux/22 -> [tpf8ac3bc8_667c_4eb5_817c_eaf14b61ea9e]
  Demux/23 -> [tpd11d2462_9c42_468f_ae22_2815283d87ec]
  Demux/24 -> [tp6fb7b211_b496_419c_a3aa_061b53cc565d]
  Demux/25 -> [tp45f0a31a_53d5_40c1_b55e_869213e25f3c]
  Demux/26 -> [tpec803859_c3c1_4941_a489_deca7022455b]
  Demux/27 -> [tp4a968b18_99c2_4604_a73a_0c59808b069d]
  Demux/28 -> [tp1313af13_b620_484c_9224_316998132f93]
  Demux/29 -> [tpe591142f_dea1_4318_96cf_203c3eb68510]
  Demux/30 -> [tpa842657a_0759_42a2_8f09_ac76eb83bf5f]
  Demux/31 -> [tpe29f236e_a886_40e5_bc3d_e445285f53b4]
  Demux/32 -> [tp9de75878_f5b7_460e_8f16_c616fc66247d]
  Demux/33 -> [tp4db8ce2b_48b9_48df_9e12_5d99a1c0522f]
  Demux/34 -> [tp4202ba58_e017_497f_a7c8_f5177773bf49]
  Demux/35 -> [tp88b394eb_2c9b_4353_a0c0_bf57c1ff4575]
  Demux/36 -> [tpb5bc6be8_b9bb_4f13_8dc4_228d35ba1bc2]
  Demux/37 -> [tp1f377af6_8adf_4d94_80d5_5b06cb5322c4]
  Demux/38 -> [tpc42da1ae_482b_4b40_95e3_7a08f1b38e38]
  Demux/39 -> [tp0482e63d_7c18_4f6a_a59c_7d531ed43ecc]
  Demux/40 -> [tp9f7021c9_dd57_458a_b060_53bd858002ca]
  Demux/41 -> [tp462c3d51_4085_4d03_922a_e7468329ecfd]
  Demux/42 -> [tp06c2d380_28df_4a86_8e1e_48fc76916ca4]
  Demux/43 -> [tpd1aa8e2b_f6fd_40c4_846e_7d350d83a9a0]
  Demux/44 -> [tp08ab0bdf_a913_447e_85cf_fffda86e9373]
  Demux/45 -> [tp226ee3c4_0555_4b6a_9dbf_0be1aa1d03cb]
  Demux/46 -> [tp5e561b6e_5b2b_4b14_a4e4_16dab790ecbc]
  Demux/47 -> [tp5917ea67_408e_4542_b440_187e98df726c]
  Demux/48 -> [tpcf20f41b_6eaf_4938_a347_e3001a381bc9]
  Demux/49 -> [tpcfe63971_5c0e_42a2_b50c_8a444b0e14b2]
  Demux/50 -> [tpb23037f8_1c1a_4214_9024_7c2fe3a041f4]
  Demux/51 -> [tp64a847ea_6418_4563_a1cf_13797fe6dc7a]
  Demux/52 -> [tpb95744bd_099f_4bff_ad66_86a571767d59]
  Demux/53 -> [tpca6fd08e_e91b_4b2c_9904_bdcc1d2b4691]
  Demux/54 -> [tpb5501c28_925b_44a1_9198_a7791897b2c3]
  Demux/55 -> [tp7ddedf46_b74b_4262_a85c_d1ae6a1a8d27]
  Demux/56 -> [tpa8a39289_d0b1_4594_a97b_af42f7bd3fbe]
  Demux/57 -> [tp0f7fa066_a738_43d7_b5ea_33fc14b95414]
  Demux/58 -> [tp12dc8a3a_3786_4253_b999_b452be1370e6]
  Demux/59 -> [tp5ba8c46d_7a0f_4206_9ccc_5b6720c2a274]
  Demux/60 -> [tpec890a5d_664b_46f4_8337_fb1cd4136c12]
  Demux/61 -> [tpf4c46696_4716_4dca_bf08_3b2d77f099fd]
  Demux/62 -> [tp4061ed8b_807e_44f2_bf58_94bd96f620e6]
  Demux/63 -> [tp9e0d15c6_2cd4_4177_8420_57047e6ecae3]
  Demux/64 -> [tp2ce8c39d_13de_4f06_b65f_37c81338e730]
  Demux/65 -> [tp3b3ecab6_ad4f_4cd3_a8fd_a37ff491354e]
  Demux/66 -> [tp866d7f9d_dc0d_43f5_9ef7_69ac0d737348]
  Demux/67 -> [tp3157eb22_59d5_477d_bce5_97fc64ee304f]
  Demux/68 -> [tpb13e888c_a9b2_4f34_ad27_7ff5b9b3ef1f]
  Demux/69 -> [tp8ce178f1_47d1_400f_a92e_b8e771fc007d]
  Demux/70 -> [tpe2e7ffdd_ab4b_4b7b_b544_448af7cdacbb]
  Demux/71 -> [tpe36d7ce5_3999_4552_94e8_e19f7995c24f]
  Demux/72 -> [tp9894fddf_c62e_4899_8e0b_28ceb3aa4861]
  Demux/73 -> [tp3718a647_e315_4173_be7d_b6524cb0e342]
  Demux/74 -> [tpf3233c60_a56c_404a_ba4c_fba2c62fb5d8]
  Demux/75 -> [tp68826778_ac3e_4c26_a61b_609335c6c26d]
  Demux/76 -> [tp81a7d01e_3be1_4270_858d_b2c6bf4b4cd2]
  Demux/77 -> [tpaa423bbf_6e7e_4fd1_a3ec_47627e81b042]
  Demux/78 -> [tp9d3c3848_08b3_49cb_b902_3b295175f898]
  Demux/79 -> [tp775764b5_8564_48a6_94cb_226c7441302a]
  Demux/80 -> [tp0c2434b1_2bab_4357_a14f_01a65cc5899d]
  Demux/81 -> [tpfb1c7bb4_efb8_4c0c_838e_88727cf4ac04]
  Demux/82 -> [tp178d29b5_8853_44aa_9b37_b50e1f7f00ee]
  Demux/83 -> [tp39c9d3df_a90b_4086_91f0_6abdae9afbf0]
  Demux/84 -> [tp4d105b44_027f_4919_9ee4_03b03b896ee0]
  Demux/85 -> [tpcec3bb7c_0484_4253_9fa8_e9c0f2ed7991]
  Demux/86 -> [tp07d5146d_e291_43b9_af20_121c131366a8]
  Demux/87 -> [tpa220758f_1834_4bc3_ae5d_4d171e25cfb0]
  Demux/88 -> [tpa24bbf75_f546_464c_a2ec_30c7c94f4878]
  Demux/89 -> [tp55580056_3bda_4be1_b974_4c33b8979e48]
  Demux/90 -> [tp73fb7770_d9f7_4ac2_8e14_684ac81fe130]
  Demux/91 -> [tp24f62f1c_7feb_4668_848a_4312b959534d]
  Demux/92 -> [tp9961bb95_9fa1_4ba6_9f00_87a6ee431af5]
  Demux/93 -> [tp3ef8d481_6f35_4e06_b3ce_eca34532af43]
  Demux/94 -> [tpf4cdafdf_c882_4bf7_af63_ac7f8207a44e]
  Demux/95 -> [tpa986df3c_0692_420a_a0e0_11daf377e2be_Va]
  Demux/96 -> [tpa986df3c_0692_420a_a0e0_11daf377e2be_Vb]
  Demux/97 -> [tpa986df3c_0692_420a_a0e0_11daf377e2be_Vc]
  Demux/98 -> [tpcc6cd470_846c_4fad_a974_bc9cf92a9d51_Va]
  Demux/99 -> [tpcc6cd470_846c_4fad_a974_bc9cf92a9d51_Vb]
  Demux/100 -> [tpcc6cd470_846c_4fad_a974_bc9cf92a9d51_Vc]
  Demux/101 -> [tpdf19fb86_054a_4874_9952_a8f14f216d53_Va]
  Demux/102 -> [tpdf19fb86_054a_4874_9952_a8f14f216d53_Vb]
  Demux/103 -> [tpdf19fb86_054a_4874_9952_a8f14f216d53_Vc]
  Demux/104 -> [tp205f070b_9a59_407e_8c0c_9150fe01e0fe_Va]
  Demux/105 -> [tp205f070b_9a59_407e_8c0c_9150fe01e0fe_Vb]
  Demux/106 -> [tp205f070b_9a59_407e_8c0c_9150fe01e0fe_Vc]
  Demux/107 -> [tp1472f817_9e66_4bc4_a0f5_ce1eea81e043_Va]
  Demux/108 -> [tp1472f817_9e66_4bc4_a0f5_ce1eea81e043_Vb]
  Demux/109 -> [tp1472f817_9e66_4bc4_a0f5_ce1eea81e043_Vc]
  Demux/110 -> [tp02ffd600_293c_4bd7_924c_5806d4af99ae_Va]
  Demux/111 -> [tp02ffd600_293c_4bd7_924c_5806d4af99ae_Vb]
  Demux/112 -> [tp02ffd600_293c_4bd7_924c_5806d4af99ae_Vc]
  Demux/113 -> [tp8826a1a8_9903_417f_9e65_9a6ae9fdba0b_Va]
  Demux/114 -> [tp8826a1a8_9903_417f_9e65_9a6ae9fdba0b_Vb]
  Demux/115 -> [tp8826a1a8_9903_417f_9e65_9a6ae9fdba0b_Vc]
  Demux/116 -> [tp9ce26310_21fc_4e2a_bc45_8aec0173af35_Va]
  Demux/117 -> [tp9ce26310_21fc_4e2a_bc45_8aec0173af35_Vb]
  Demux/118 -> [tp9ce26310_21fc_4e2a_bc45_8aec0173af35_Vc]
  Demux/119 -> [tp5c3ec21a_2446_4a93_86fa_50167eb0bb49_Va]
  Demux/120 -> [tp5c3ec21a_2446_4a93_86fa_50167eb0bb49_Vb]
  Demux/121 -> [tp5c3ec21a_2446_4a93_86fa_50167eb0bb49_Vc]
  Demux/122 -> [tp6feed814_e1fc_4ccc_aee1_0f1dbac7f21c_Va]
  Demux/123 -> [tp6feed814_e1fc_4ccc_aee1_0f1dbac7f21c_Vb]
  Demux/124 -> [tp6feed814_e1fc_4ccc_aee1_0f1dbac7f21c_Vc]
  Demux/125 -> [tp47961249_9827_46c9_8df4_4332c0d936a6_Va]
  Demux/126 -> [tp47961249_9827_46c9_8df4_4332c0d936a6_Vb]
  Demux/127 -> [tp47961249_9827_46c9_8df4_4332c0d936a6_Vc]
  Demux/128 -> [tp0a524b2c_b8aa_44b5_8af1_83103f6fe7fa_Va]
  Demux/129 -> [tp0a524b2c_b8aa_44b5_8af1_83103f6fe7fa_Vb]
  Demux/130 -> [tp0a524b2c_b8aa_44b5_8af1_83103f6fe7fa_Vc]
  Demux/131 -> [tpe68302e0_d7cc_4cde_9e4d_d65be10fe8ce_Va]
  Demux/132 -> [tpe68302e0_d7cc_4cde_9e4d_d65be10fe8ce_Vb]
  Demux/133 -> [tpe68302e0_d7cc_4cde_9e4d_d65be10fe8ce_Vc]
  Demux/134 -> [tpb6741d7e_7104_42f6_b202_2624712a66dd_Va]
  Demux/135 -> [tpb6741d7e_7104_42f6_b202_2624712a66dd_Vb]
  Demux/136 -> [tpb6741d7e_7104_42f6_b202_2624712a66dd_Vc]
  Demux/137 -> [tpf1aac363_9296_4953_add4_e120d0d16a9c_Va]
  Demux/138 -> [tpf1aac363_9296_4953_add4_e120d0d16a9c_Vb]
  Demux/139 -> [tpf1aac363_9296_4953_add4_e120d0d16a9c_Vc]
  Demux/140 -> [tp887a83b4_1d25_4153_8696_aa60dda32590_Va]
  Demux/141 -> [tp887a83b4_1d25_4153_8696_aa60dda32590_Vb]
  Demux/142 -> [tp887a83b4_1d25_4153_8696_aa60dda32590_Vc]
  Demux/143 -> [tp525020f9_0518_43bd_bd08_395cececd30f_Va]
  Demux/144 -> [tp525020f9_0518_43bd_bd08_395cececd30f_Vb]
  Demux/145 -> [tp525020f9_0518_43bd_bd08_395cececd30f_Vc]
  Demux/146 -> [tp07e0d3ab_a036_409a_85fb_5d4a0c03bed4_Va]
  Demux/147 -> [tp07e0d3ab_a036_409a_85fb_5d4a0c03bed4_Vb]
  Demux/148 -> [tp07e0d3ab_a036_409a_85fb_5d4a0c03bed4_Vc]
  Demux/149 -> [tpfcaa7117_49ae_495f_adc8_59d0c6f9f67d_Va]
  Demux/150 -> [tpfcaa7117_49ae_495f_adc8_59d0c6f9f67d_Vb]
  Demux/151 -> [tpfcaa7117_49ae_495f_adc8_59d0c6f9f67d_Vc]
  Demux/152 -> [tp31eb8ead_2d59_483a_bca9_f86ed99f91ce_Va]
  Demux/153 -> [tp31eb8ead_2d59_483a_bca9_f86ed99f91ce_Vb]
  Demux/154 -> [tp31eb8ead_2d59_483a_bca9_f86ed99f91ce_Vc]
  Demux/155 -> [tpe179a349_ae85_4693_8cd0_995eb2e043ad_Va]
  Demux/156 -> [tpe179a349_ae85_4693_8cd0_995eb2e043ad_Vb]
  Demux/157 -> [tpe179a349_ae85_4693_8cd0_995eb2e043ad_Vc]
  Demux/158 -> [tpce2fb862_6c96_4958_bb93_fa141764bed3_Va]
  Demux/159 -> [tpce2fb862_6c96_4958_bb93_fa141764bed3_Vb]
  Demux/160 -> [tpce2fb862_6c96_4958_bb93_fa141764bed3_Vc]
  Demux/161 -> [tp88ce0a48_0233_47ea_86c8_f79f90af2cd6_Va]
  Demux/162 -> [tp88ce0a48_0233_47ea_86c8_f79f90af2cd6_Vb]
  Demux/163 -> [tp88ce0a48_0233_47ea_86c8_f79f90af2cd6_Vc]
  Demux/164 -> [tpd11d9ec5_c08b_4d96_8652_f0f49e420851_Va]
  Demux/165 -> [tpd11d9ec5_c08b_4d96_8652_f0f49e420851_Vb]
  Demux/166 -> [tpd11d9ec5_c08b_4d96_8652_f0f49e420851_Vc]
  Demux/167 -> [tp23d930d0_b85e_4ceb_9e3a_12c30c008bc7_Va]
  Demux/168 -> [tp23d930d0_b85e_4ceb_9e3a_12c30c008bc7_Vb]
  Demux/169 -> [tp23d930d0_b85e_4ceb_9e3a_12c30c008bc7_Vc]
  Demux/170 -> [tp9c4b3537_3589_46e6_9553_b363e3b9b752_Va]
  Demux/171 -> [tp9c4b3537_3589_46e6_9553_b363e3b9b752_Vb]
  Demux/172 -> [tp9c4b3537_3589_46e6_9553_b363e3b9b752_Vc]
  Demux/173 -> [tp1dbfb037_9537_4d7d_a599_453ac64101ac_Va]
  Demux/174 -> [tp1dbfb037_9537_4d7d_a599_453ac64101ac_Vb]
  Demux/175 -> [tp1dbfb037_9537_4d7d_a599_453ac64101ac_Vc]
  Demux/176 -> [tp54ea34e2_243f_4702_ac79_9d927b1519bb_Va]
  Demux/177 -> [tp54ea34e2_243f_4702_ac79_9d927b1519bb_Vb]
  Demux/178 -> [tp54ea34e2_243f_4702_ac79_9d927b1519bb_Vc]
  Demux/179 -> [tp2c67bf33_0d47_4572_bd34_923d279308e1_Va]
  Demux/180 -> [tp2c67bf33_0d47_4572_bd34_923d279308e1_Vb]
  Demux/181 -> [tp2c67bf33_0d47_4572_bd34_923d279308e1_Vc]
  Demux/182 -> [tpb9c0cf8e_1902_4be0_b38c_875a34200abd_Va]
  Demux/183 -> [tpb9c0cf8e_1902_4be0_b38c_875a34200abd_Vb]
  Demux/184 -> [tpb9c0cf8e_1902_4be0_b38c_875a34200abd_Vc]
  Demux/185 -> [tp03542e2a_7fe7_437d_8550_cad07cd34d13_Va]
  Demux/186 -> [tp03542e2a_7fe7_437d_8550_cad07cd34d13_Vb]
  Demux/187 -> [tp03542e2a_7fe7_437d_8550_cad07cd34d13_Vc]
  Demux/188 -> [tpb67c8fd4_0a32_4203_afab_338e2927144e_Va]
  Demux/189 -> [tpb67c8fd4_0a32_4203_afab_338e2927144e_Vb]
  Demux/190 -> [tpb67c8fd4_0a32_4203_afab_338e2927144e_Vc]
  Demux/191 -> [tp1c80e86a_0d31_411c_9f65_09f5514ae1cb_Va]
  Demux/192 -> [tp1c80e86a_0d31_411c_9f65_09f5514ae1cb_Vb]
  Demux/193 -> [tp1c80e86a_0d31_411c_9f65_09f5514ae1cb_Vc]
  Demux/194 -> [tp0a6ed6e3_d61a_499f_b0b2_92e278c8b95c_Va]
  Demux/195 -> [tp0a6ed6e3_d61a_499f_b0b2_92e278c8b95c_Vb]
  Demux/196 -> [tp0a6ed6e3_d61a_499f_b0b2_92e278c8b95c_Vc]
  Demux/197 -> [tpf963f17b_f1b4_4eb9_9f2c_2e7f4c8c923d_Va]
  Demux/198 -> [tpf963f17b_f1b4_4eb9_9f2c_2e7f4c8c923d_Vb]
  Demux/199 -> [tpf963f17b_f1b4_4eb9_9f2c_2e7f4c8c923d_Vc]
  Demux/200 -> [tp43e10b86_c8d4_46ca_9a46_1b5c8c9df653_Va]

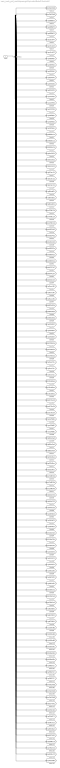
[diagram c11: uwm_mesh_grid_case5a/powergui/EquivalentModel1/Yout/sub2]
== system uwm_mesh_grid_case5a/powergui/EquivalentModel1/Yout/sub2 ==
  input : Inport  OutDataType=sfix(16)  OutScaling=2^0
  Demux : Demux  Outputs=[1 1 1 1 1 1 1 1 1 1 1 1 1 1 1 1 1 1 1 1 1 1 1 1 1 1 1 1 1 1 1 1 1 1 1 1 1 1 1 1 1 1 1 1 1 1 1 1 1 1 1 1 1 1 1 1 1 1 1 1 1 1 1 1 1 1 1 1 1 1 1 1 1 1 1 1 1 1 1 1 1 1 1 1 1 1 1 1 1 1 1 1 1 1 1 1 1 1 1 1 1 1 1 1 1 1 1 1 1 1 1 1 1 1 1 1 1 1 1 1]
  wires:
  input/1 -> Demux/1
  Demux/1 -> [tp43e10b86_c8d4_46ca_9a46_1b5c8c9df653_Vb]
  Demux/2 -> [tp43e10b86_c8d4_46ca_9a46_1b5c8c9df653_Vc]
  Demux/3 -> [tpa986df3c_0692_420a_a0e0_11daf377e2be_Ia]
  Demux/4 -> [tpa986df3c_0692_420a_a0e0_11daf377e2be_Ib]
  Demux/5 -> [tpa986df3c_0692_420a_a0e0_11daf377e2be_Ic]
  Demux/6 -> [tpcc6cd470_846c_4fad_a974_bc9cf92a9d51_Ia]
  Demux/7 -> [tpcc6cd470_846c_4fad_a974_bc9cf92a9d51_Ib]
  Demux/8 -> [tpcc6cd470_846c_4fad_a974_bc9cf92a9d51_Ic]
  Demux/9 -> [tpdf19fb86_054a_4874_9952_a8f14f216d53_Ia]
  Demux/10 -> [tpdf19fb86_054a_4874_9952_a8f14f216d53_Ib]
  Demux/11 -> [tpdf19fb86_054a_4874_9952_a8f14f216d53_Ic]
  Demux/12 -> [tp205f070b_9a59_407e_8c0c_9150fe01e0fe_Ia]
  Demux/13 -> [tp205f070b_9a59_407e_8c0c_9150fe01e0fe_Ib]
  Demux/14 -> [tp205f070b_9a59_407e_8c0c_9150fe01e0fe_Ic]
  Demux/15 -> [tp1472f817_9e66_4bc4_a0f5_ce1eea81e043_Ia]
  Demux/16 -> [tp1472f817_9e66_4bc4_a0f5_ce1eea81e043_Ib]
  Demux/17 -> [tp1472f817_9e66_4bc4_a0f5_ce1eea81e043_Ic]
  Demux/18 -> [tp02ffd600_293c_4bd7_924c_5806d4af99ae_Ia]
  Demux/19 -> [tp02ffd600_293c_4bd7_924c_5806d4af99ae_Ib]
  Demux/20 -> [tp02ffd600_293c_4bd7_924c_5806d4af99ae_Ic]
  Demux/21 -> [tp8826a1a8_9903_417f_9e65_9a6ae9fdba0b_Ia]
  Demux/22 -> [tp8826a1a8_9903_417f_9e65_9a6ae9fdba0b_Ib]
  Demux/23 -> [tp8826a1a8_9903_417f_9e65_9a6ae9fdba0b_Ic]
  Demux/24 -> [tp9ce26310_21fc_4e2a_bc45_8aec0173af35_Ia]
  Demux/25 -> [tp9ce26310_21fc_4e2a_bc45_8aec0173af35_Ib]
  Demux/26 -> [tp9ce26310_21fc_4e2a_bc45_8aec0173af35_Ic]
  Demux/27 -> [tp5c3ec21a_2446_4a93_86fa_50167eb0bb49_Ia]
  Demux/28 -> [tp5c3ec21a_2446_4a93_86fa_50167eb0bb49_Ib]
  Demux/29 -> [tp5c3ec21a_2446_4a93_86fa_50167eb0bb49_Ic]
  Demux/30 -> [tp6feed814_e1fc_4ccc_aee1_0f1dbac7f21c_Ia]
  Demux/31 -> [tp6feed814_e1fc_4ccc_aee1_0f1dbac7f21c_Ib]
  Demux/32 -> [tp6feed814_e1fc_4ccc_aee1_0f1dbac7f21c_Ic]
  Demux/33 -> [tp47961249_9827_46c9_8df4_4332c0d936a6_Ia]
  Demux/34 -> [tp47961249_9827_46c9_8df4_4332c0d936a6_Ib]
  Demux/35 -> [tp47961249_9827_46c9_8df4_4332c0d936a6_Ic]
  Demux/36 -> [tp0a524b2c_b8aa_44b5_8af1_83103f6fe7fa_Ia]
  Demux/37 -> [tp0a524b2c_b8aa_44b5_8af1_83103f6fe7fa_Ib]
  Demux/38 -> [tp0a524b2c_b8aa_44b5_8af1_83103f6fe7fa_Ic]
  Demux/39 -> [tpe68302e0_d7cc_4cde_9e4d_d65be10fe8ce_Ia]
  Demux/40 -> [tpe68302e0_d7cc_4cde_9e4d_d65be10fe8ce_Ib]
  Demux/41 -> [tpe68302e0_d7cc_4cde_9e4d_d65be10fe8ce_Ic]
  Demux/42 -> [tpb6741d7e_7104_42f6_b202_2624712a66dd_Ia]
  Demux/43 -> [tpb6741d7e_7104_42f6_b202_2624712a66dd_Ib]
  Demux/44 -> [tpb6741d7e_7104_42f6_b202_2624712a66dd_Ic]
  Demux/45 -> [tpf1aac363_9296_4953_add4_e120d0d16a9c_Ia]
  Demux/46 -> [tpf1aac363_9296_4953_add4_e120d0d16a9c_Ib]
  Demux/47 -> [tpf1aac363_9296_4953_add4_e120d0d16a9c_Ic]
  Demux/48 -> [tp887a83b4_1d25_4153_8696_aa60dda32590_Ia]
  Demux/49 -> [tp887a83b4_1d25_4153_8696_aa60dda32590_Ib]
  Demux/50 -> [tp887a83b4_1d25_4153_8696_aa60dda32590_Ic]
  Demux/51 -> [tp525020f9_0518_43bd_bd08_395cececd30f_Ia]
  Demux/52 -> [tp525020f9_0518_43bd_bd08_395cececd30f_Ib]
  Demux/53 -> [tp525020f9_0518_43bd_bd08_395cececd30f_Ic]
  Demux/54 -> [tp07e0d3ab_a036_409a_85fb_5d4a0c03bed4_Ia]
  Demux/55 -> [tp07e0d3ab_a036_409a_85fb_5d4a0c03bed4_Ib]
  Demux/56 -> [tp07e0d3ab_a036_409a_85fb_5d4a0c03bed4_Ic]
  Demux/57 -> [tpfcaa7117_49ae_495f_adc8_59d0c6f9f67d_Ia]
  Demux/58 -> [tpfcaa7117_49ae_495f_adc8_59d0c6f9f67d_Ib]
  Demux/59 -> [tpfcaa7117_49ae_495f_adc8_59d0c6f9f67d_Ic]
  Demux/60 -> [tp31eb8ead_2d59_483a_bca9_f86ed99f91ce_Ia]
  Demux/61 -> [tp31eb8ead_2d59_483a_bca9_f86ed99f91ce_Ib]
  Demux/62 -> [tp31eb8ead_2d59_483a_bca9_f86ed99f91ce_Ic]
  Demux/63 -> [tpe179a349_ae85_4693_8cd0_995eb2e043ad_Ia]
  Demux/64 -> [tpe179a349_ae85_4693_8cd0_995eb2e043ad_Ib]
  Demux/65 -> [tpe179a349_ae85_4693_8cd0_995eb2e043ad_Ic]
  Demux/66 -> [tpce2fb862_6c96_4958_bb93_fa141764bed3_Ia]
  Demux/67 -> [tpce2fb862_6c96_4958_bb93_fa141764bed3_Ib]
  Demux/68 -> [tpce2fb862_6c96_4958_bb93_fa141764bed3_Ic]
  Demux/69 -> [tp88ce0a48_0233_47ea_86c8_f79f90af2cd6_Ia]
  Demux/70 -> [tp88ce0a48_0233_47ea_86c8_f79f90af2cd6_Ib]
  Demux/71 -> [tp88ce0a48_0233_47ea_86c8_f79f90af2cd6_Ic]
  Demux/72 -> [tpd11d9ec5_c08b_4d96_8652_f0f49e420851_Ia]
  Demux/73 -> [tpd11d9ec5_c08b_4d96_8652_f0f49e420851_Ib]
  Demux/74 -> [tpd11d9ec5_c08b_4d96_8652_f0f49e420851_Ic]
  Demux/75 -> [tp23d930d0_b85e_4ceb_9e3a_12c30c008bc7_Ia]
  Demux/76 -> [tp23d930d0_b85e_4ceb_9e3a_12c30c008bc7_Ib]
  Demux/77 -> [tp23d930d0_b85e_4ceb_9e3a_12c30c008bc7_Ic]
  Demux/78 -> [tp9c4b3537_3589_46e6_9553_b363e3b9b752_Ia]
  Demux/79 -> [tp9c4b3537_3589_46e6_9553_b363e3b9b752_Ib]
  Demux/80 -> [tp9c4b3537_3589_46e6_9553_b363e3b9b752_Ic]
  Demux/81 -> [tp1dbfb037_9537_4d7d_a599_453ac64101ac_Ia]
  Demux/82 -> [tp1dbfb037_9537_4d7d_a599_453ac64101ac_Ib]
  Demux/83 -> [tp1dbfb037_9537_4d7d_a599_453ac64101ac_Ic]
  Demux/84 -> [tp54ea34e2_243f_4702_ac79_9d927b1519bb_Ia]
  Demux/85 -> [tp54ea34e2_243f_4702_ac79_9d927b1519bb_Ib]
  Demux/86 -> [tp54ea34e2_243f_4702_ac79_9d927b1519bb_Ic]
  Demux/87 -> [tp2c67bf33_0d47_4572_bd34_923d279308e1_Ia]
  Demux/88 -> [tp2c67bf33_0d47_4572_bd34_923d279308e1_Ib]
  Demux/89 -> [tp2c67bf33_0d47_4572_bd34_923d279308e1_Ic]
  Demux/90 -> [tpb9c0cf8e_1902_4be0_b38c_875a34200abd_Ia]
  Demux/91 -> [tpb9c0cf8e_1902_4be0_b38c_875a34200abd_Ib]
  Demux/92 -> [tpb9c0cf8e_1902_4be0_b38c_875a34200abd_Ic]
  Demux/93 -> [tp03542e2a_7fe7_437d_8550_cad07cd34d13_Ia]
  Demux/94 -> [tp03542e2a_7fe7_437d_8550_cad07cd34d13_Ib]
  Demux/95 -> [tp03542e2a_7fe7_437d_8550_cad07cd34d13_Ic]
  Demux/96 -> [tpb67c8fd4_0a32_4203_afab_338e2927144e_Ia]
  Demux/97 -> [tpb67c8fd4_0a32_4203_afab_338e2927144e_Ib]
  Demux/98 -> [tpb67c8fd4_0a32_4203_afab_338e2927144e_Ic]
  Demux/99 -> [tp1c80e86a_0d31_411c_9f65_09f5514ae1cb_Ia]
  Demux/100 -> [tp1c80e86a_0d31_411c_9f65_09f5514ae1cb_Ib]
  Demux/101 -> [tp1c80e86a_0d31_411c_9f65_09f5514ae1cb_Ic]
  Demux/102 -> [tp0a6ed6e3_d61a_499f_b0b2_92e278c8b95c_Ia]
  Demux/103 -> [tp0a6ed6e3_d61a_499f_b0b2_92e278c8b95c_Ib]
  Demux/104 -> [tp0a6ed6e3_d61a_499f_b0b2_92e278c8b95c_Ic]
  Demux/105 -> [tpf963f17b_f1b4_4eb9_9f2c_2e7f4c8c923d_Ia]
  Demux/106 -> [tpf963f17b_f1b4_4eb9_9f2c_2e7f4c8c923d_Ib]
  Demux/107 -> [tpf963f17b_f1b4_4eb9_9f2c_2e7f4c8c923d_Ic]
  Demux/108 -> [tp43e10b86_c8d4_46ca_9a46_1b5c8c9df653_Ia]
  Demux/109 -> [tp43e10b86_c8d4_46ca_9a46_1b5c8c9df653_Ib]
  Demux/110 -> [tp43e10b86_c8d4_46ca_9a46_1b5c8c9df653_Ic]
  Demux/111 -> [tpd2c7d01d_327d_4af0_a76f_8d9568e59706]
  Demux/112 -> [tp1c6d1dd1_e6dd_4875_b87b_8d3009847d3d]
  Demux/113 -> [tp87a437f7_95ba_446a_92b4_e61fb294ff49]
  Demux/114 -> [tpd3f1e11d_605c_483c_9381_1a5c30855e07]
  Demux/115 -> [tp38130af3_d2c8_4768_94af_2d9c3b941f09]
  Demux/116 -> [tp6657681e_ded5_42db_9df9_ab5bd56ccc9e]
  Demux/117 -> [tpd5881c92_0758_406d_814c_0355fd984bcf]
  Demux/118 -> [tpc9543e37_d500_497d_a150_fe1094b8d930]
  Demux/119 -> [tp1033c174_81cb_42aa_93db_e3a5a988fd0f]
  Demux/120 -> [tp70ce9907_09f9_4605_be9e_ede5c090b291]
